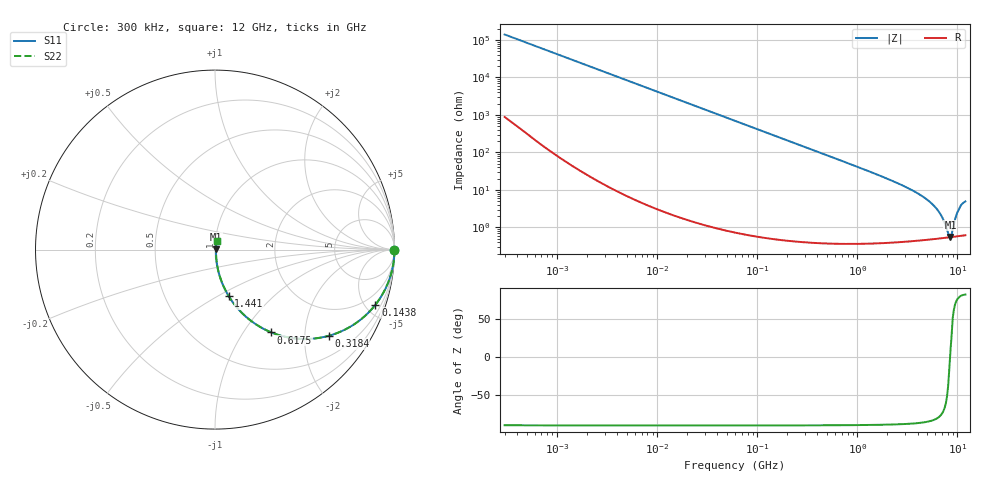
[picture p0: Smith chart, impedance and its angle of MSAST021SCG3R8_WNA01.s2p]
! MSAST021SCG3R8_WNA01  S-PARAMETER MODEL  ( General Type )
! Model Generated by TAIYO YUDEN Corporation (http://www.ty-top.com)
! Version 2.0
! TAIYO YUDEN Control No. 181101
! Copyright(c) 2015 TAIYO YUDEN CO.,LTD. All Rights Reserved.
! Product Description (link to TY-COMPAS)
! https://ds.yuden.co.jp/TYCOMPAS/or/detail?pn=MSAST021SCG3R8BWNA01&u=M
! Products Name : Multilayer Ceramic Capacitors
! Characteristics :
!  Capacitance : 3.8 pF , Rated Voltage : 25V , TCC : CG / C0G
!  Case Size : 0.25 x 0.125 / 0.0098 x 0.0049 [mm/inch] , Thickness : 0.125 / 0.0049 [mm/inch]
!  (Conditions: Temperature = 25 degC , DC Bias Current/Voltage = 0A / 0V)
! External Node Assignments :
!  1  o---| |---o  2
! GND o---------o GND
! Frequency Range : 0.3MHz  -  12000MHz  [ 401 STEP ]
# MHz S RI R 50
! Freq[MHz].  S11 Real  S11 Imag  S21 Real  S21 Imag  S12 Real  S12 Imag  S22 Real  S22 Imag
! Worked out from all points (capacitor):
!   401 points, 300 kHz to 12 GHz, reference 50 ohm
!   read as one part in series: C = 3.8 pF near 316.3 kHz
!   lowest |Z| = 553 mohm at 8.504 GHz (marker M1)
!   series resonance near 8.433 GHz, so ESL is about 94 pH
!   S11 on the Smith chart (normalised r, x): 300 kHz: open; 143.8 MHz: 1.01, -5.82; 318.4 MHz: 1.01, -2.63; 617.5 MHz: 1.01, -1.35; 1.441 GHz: 1.01, -0.56; 12 GHz: 1.01, +0.10
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0.3  1 -0.000716  5.04e-06 0.000716  5.04e-06 0.000716  1 -0.000716
1.769972  1 -0.00423  2.33e-05 0.00423  2.33e-05 0.00423  1 -0.00423
10.44266  0.9994 -0.0249  0.000639 0.0249  0.000639 0.0249  0.9994 -0.0249
60  0.9797 -0.1403  0.0203 0.1403  0.0203 0.1403  0.9797 -0.1403
143.8206  0.8941 -0.3069  0.1059 0.3069  0.1059 0.3069  0.8941 -0.3069
318.4019  0.6327 -0.4806  0.3673 0.4806  0.3673 0.4806  0.6327 -0.4806
353.9943  0.5822 -0.4916  0.4178 0.4916  0.4178 0.4916  0.5822 -0.4916
617.4538  0.3137 -0.4613  0.6863 0.4613  0.6863 0.4613  0.3137 -0.4613
943.3804  0.1633 -0.3655  0.8367 0.3655  0.8367 0.3655  0.1633 -0.3655
1441.349  0.0766 -0.2595  0.9234 0.2595  0.9234 0.2595  0.0766 -0.2595
2088.533  0.0377 -0.1804  0.9623 0.1804  0.9623 0.1804  0.0377 -0.1804
3740.715  0.0122 -0.0884  0.9878 0.0884  0.9878 0.0884  0.0122 -0.0884
5420.343  0.00676 -0.0447  0.9932 0.0447  0.9932 0.0447  0.00676 -0.0447
6699.894  0.00557 -0.0226  0.9944 0.0226  0.9944 0.0226  0.00557 -0.0226
7254.098  0.00539 -0.0147  0.9946 0.0147  0.9946 0.0147  0.00539 -0.0147
8064.993  0.00537 -0.00419  0.9946 0.00419  0.9946 0.00419  0.00537 -0.00419
8503.825  0.00545 0.000729  0.9945 -0.000729  0.9945 -0.000729  0.00545 0.000729
8732.115  0.00551 0.00292  0.9945 -0.00292  0.9945 -0.00292  0.00551 0.00292
9708.23  0.00609 0.0197  0.9939 -0.0197  0.9939 -0.0197  0.00609 0.0197
10236.47  0.00659 0.028  0.9934 -0.028  0.9934 -0.028  0.00659 0.028
11083.22  0.00765 0.0409  0.9924 -0.0409  0.9924 -0.0409  0.00765 0.0409
12000  0.00847 0.0481  0.9915 -0.0481  0.9915 -0.0481  0.00847 0.0481
